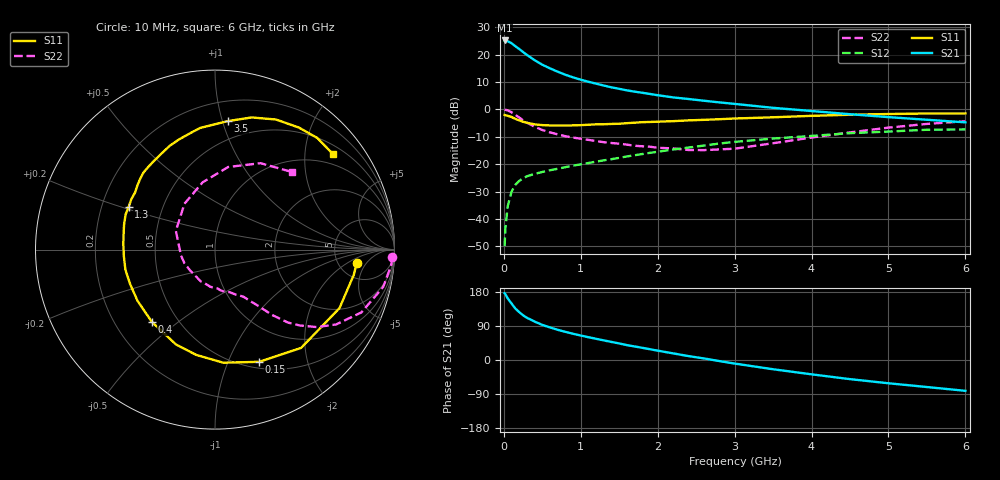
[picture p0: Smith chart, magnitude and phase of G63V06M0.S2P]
! SIEMENS Small Signal Semiconductors
! BFG193
! Si NPN RF Bipolar Junction Transistor in SOT223
! VCE = 3 V  IC = 6 mA
! Common Emitter S-Parameters:  August  1996
# GHz  S  MA  R  50
!  f  S11  S21  S12  S22
! GHz  MAG  ANG  MAG  ANG  MAG  ANG  MAG  ANG
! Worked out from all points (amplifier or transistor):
!   36 points, 10 MHz to 6 GHz, reference 50 ohm
!   highest |S21| = 25.2 dB at 10 MHz (marker M1)
!   |S21| within 3 dB of that: start of sweep to 193.8 MHz
!   unconditionally stable (mu >= 1): 1.042 GHz to 2.589 GHz
!   at 250 MHz: K = 0.39, MSG = 23.0 dB, |S12| = -25.1 dB
!   at 1.4 GHz: K = 1.09, MAG = 11.3 dB, |S12| = -18.1 dB
!   at 6 GHz: K = 0.89, MSG = 1.3 dB, |S12| = -7.3 dB
!   S11 on the Smith chart (normalised r, x): 10 MHz: 7.48, -2.95; 150 MHz: 0.57, -1.30; 400 MHz: 0.36, -0.40; 1.3 GHz: 0.32, +0.21; 3.5 GHz: 0.35, +1.04; 6 GHz: 0.71, +2.65
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0.01  0.7929 -5.3  18.14 176.3  0.0032 88.7  0.9895 -2.5
0.02  0.786 -10.3  18.07 173.8  0.0067 84.3  0.9853 -5.1
0.05  0.7663 -25.2  17.55 162.7  0.0171 77.9  0.9601 -12.5
0.1  0.7281 -48.8  16.16 149.1  0.0315 67.7  0.8879 -23.2
0.15  0.6719 -68.5  14.24 135.7  0.0423 57.9  0.7936 -31.7
0.2  0.6319 -85.8  12.65 126.4  0.0497 53.3  0.7123 -37.3
0.25  0.596 -100.1  11.16 117.9  0.0555 48.6  0.6326 -41.9
0.3  0.5715 -112.4  9.873 111.4  0.0604 46.2  0.5748 -45.0
0.4  0.5346 -131.2  7.935 101.4  0.0666 42.7  0.4828 -48.9
0.5  0.5175 -146.5  6.547 92.6  0.0723 41.0  0.4221 -51.2
0.6  0.5106 -158.0  5.61 85.9  0.0777 40.9  0.3812 -53.3
0.7  0.5115 -167.4  4.885 79.7  0.0827 41.3  0.3508 -55.4
0.9  0.5118 176.4  3.847 69.2  0.0944 41.2  0.3065 -58.9
1.1  0.5255 164.6  3.194 60.1  0.1053 41.5  0.2782 -64.9
1.3  0.5366 153.8  2.729 51.7  0.118 41.1  0.2524 -70.5
1.6  0.5616 140.3  2.229 39.3  0.1389 39.4  0.2279 -82.6
2.2  0.6113 119.6  1.659 17.5  0.1856 32.5  0.1945 -113.7
2.8  0.6633 102.0  1.346 -2.8  0.2384 22.6  0.1864 -155.8
3.5  0.7191 84.4  1.07 -24.4  0.2942 7.3  0.2418 154.4
4.5  0.8004 64.9  0.818 -50.5  0.369 -13.0  0.3812 100.4
5.5  0.8436 47.5  0.648 -71.3  0.4257 -38.2  0.5443 62.2
6  0.8455 39.1  0.581 -81.4  0.4321 -52.5  0.609 45.2
